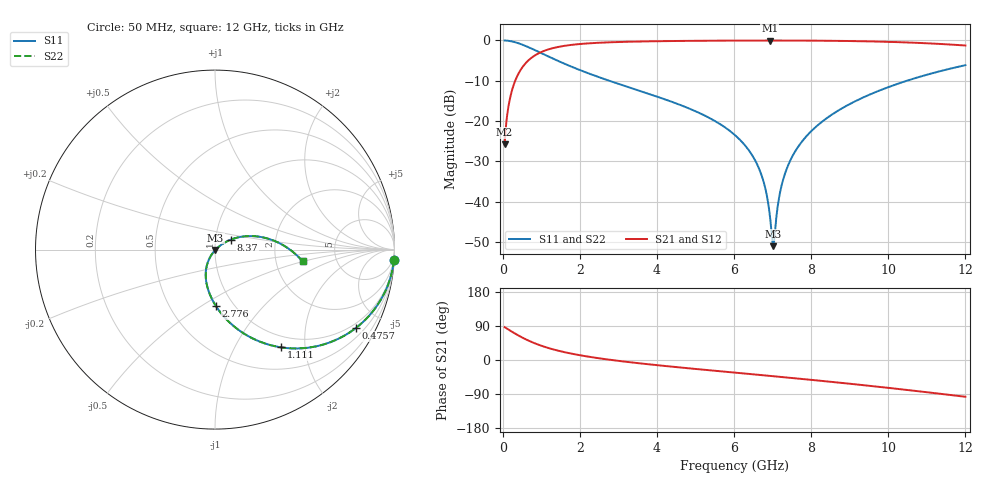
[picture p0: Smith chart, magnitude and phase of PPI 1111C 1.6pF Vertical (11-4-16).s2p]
# GHz S MA R 50
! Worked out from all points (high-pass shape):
!   1601 points, 50 MHz to 12 GHz, reference 50 ohm
!   highest |S21| = -0.03 dB at 6.929 GHz (marker M1); lowest = -25.8 dB at 50 MHz (marker M2)
!   |S21| within 3 dB of the highest: 968.4 MHz to end of sweep
!   lowest |S11| = -51.0 dB at 7.018 GHz (marker M3), VSWR 1.01, Z = 50.2 - j0.181 ohm
!   |S11| at or under -10 dB: 2.761 GHz to 10.49 GHz (7.725 GHz wide, 117 % of centre)
!   |S22| runs from -51.0 to 0.0 dB; largest |S21 - S12| = 0
!   S11 on the Smith chart (normalised r, x): 50 MHz: 1, -35; 475.7 MHz: 0.81, -3.69; 1.111 GHz: 0.82, -1.56; 2.776 GHz: 0.83, -0.58; 8.37 GHz: 1.19, +0.13; 12 GHz: 2.85, -0.49
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0.05  0.9987 -3.3  0.05117 86.7  0.05117 86.7  0.9987 -3.3
0.2217813  0.9751 -14.2  0.2217 75.8  0.2217 75.8  0.9751 -14.2
0.4757188  0.8985 -29.1  0.4385 60.9  0.4385 60.9  0.8985 -29.1
1.110562  0.6571 -56.0  0.7528 34.0  0.7528 34.0  0.6571 -56.0
2.044156  0.4211 -78.0  0.9056 11.8  0.9056 11.8  0.4211 -78.0
2.776094  0.3144 -89.1  0.9476 0.7  0.9476 0.7  0.3144 -89.1
4.038312  0.1982 -103.5  0.9781 -14.0  0.9781 -14.0  0.1982 -103.5
5.24825  0.1163 -114.9  0.9907 -26.0  0.9907 -26.0  0.1163 -114.9
6.025  0.06677 -121.3  0.995 -33.4  0.995 -33.4  0.06677 -121.3
6.637437  0.02641 -123.4  0.9966 -39.1  0.9966 -39.1  0.02641 -123.4
6.809219  0.01476 -120.2  0.9968 -40.8  0.9968 -40.8  0.01476 -120.2
6.928719  0.006772 -107.8  0.9968 -41.9  0.9968 -41.9  0.006772 -107.8
6.981  0.003745 -84.4  0.9968 -42.4  0.9968 -42.4  0.003745 -84.4
7.018344  0.002802 -40.0  0.9968 -42.8  0.9968 -42.8  0.002802 -40.0
7.055688  0.003964 1.7  0.9968 -43.1  0.9968 -43.1  0.003964 1.7
7.190125  0.01278 32.6  0.9967 -44.4  0.9967 -44.4  0.01278 32.6
7.354438  0.02467 37.2  0.9964 -46.0  0.9964 -46.0  0.02467 37.2
7.630781  0.04546 37.5  0.9955 -48.7  0.9955 -48.7  0.04546 37.5
8.019156  0.0762 35.0  0.9935 -52.5  0.9935 -52.5  0.0762 35.0
8.370188  0.1056 32.1  0.9906 -56.1  0.9906 -56.1  0.1056 32.1
10.01331  0.2644 15.5  0.9597 -73.6  0.9597 -73.6  0.2644 15.5
12  0.4928 -7.6  0.8643 -97.0  0.8643 -97.0  0.4928 -7.6
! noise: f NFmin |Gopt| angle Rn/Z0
0.05  0.0007563  0.9532  2.214  0.003636
1.372  0.004072  0.7004  11.42  0.002635
2.701  0.006393  0.6395  19.21  0.003259
4.031  0.008485  0.6101  26.86  0.003829
5.36  0.01052  0.5974  34.19  0.004416
6.682  0.01258  0.5964  41.08  0.005068
8.012  0.01477  0.6042  47.57  0.005839
9.341  0.01715  0.6192  53.64  0.006782
10.67  0.01982  0.6401  59.33  0.007974
12  0.02288  0.6657  64.71  0.009517
